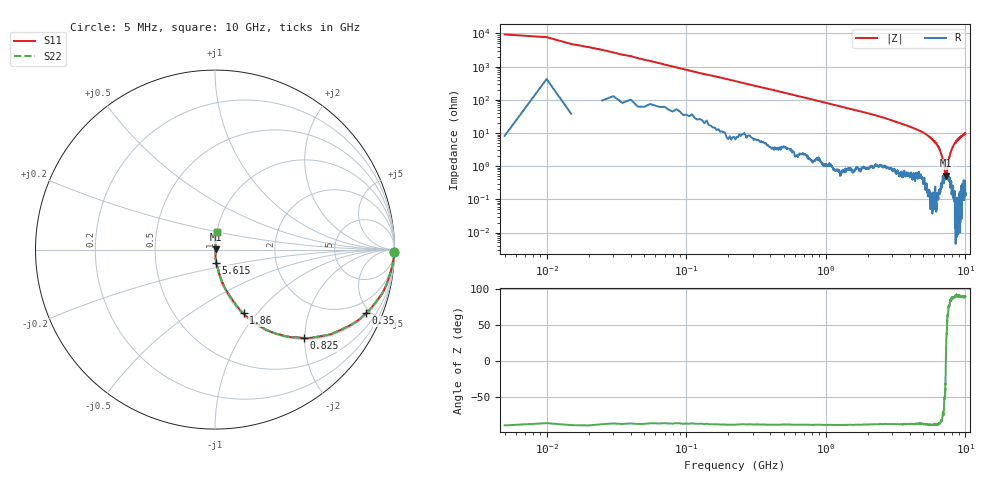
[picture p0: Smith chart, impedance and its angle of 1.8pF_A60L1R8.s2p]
! Amotech Co.,Ltd.
! http://www.amotech.co.kr/
! Part Number: A60L1R8
! These Parameters are Measured in Series Mode Connection
! Operation Temp=25[degC], DC Bias Voltage=0[V]
! Freq. Start=5[MHz] Stop=10[GHz], 2000[Steps]
! Date: Monday, July 14, 2020, 09:28:34
# GHZ S RI R 50.000000
!Freq.(Hz) S11(Real) S11(Imag) S21(Real) S21(Imag) S12(Real) S12(Imag) S22(Real) S22(Imag)
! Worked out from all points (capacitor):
!   2000 points, 5 MHz to 10 GHz, reference 50 ohm
!   read as one part in series: C = 1.98 pF near 55 MHz
!   lowest |Z| = 519 mohm at 7.28 GHz (marker M1)
!   series resonance near 7.248 GHz, so ESL is about 240 pH
!   S11 on the Smith chart (normalised r, x): 5 MHz: open; 350 MHz: 1.10, -4.72; 825 MHz: 1.03, -1.98; 1.86 GHz: 1.02, -0.85; 5.615 GHz: 1.00, -0.15; 10 GHz: 1.00, +0.20
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0.005  0.9999 -0.0107  0.000124 0.0107  0.000124 0.0107  0.9999 -0.0107
0.07  0.9881 -0.0851  0.0119 0.0851  0.0119 0.0851  0.9881 -0.0851
0.12  0.9728 -0.1447  0.0272 0.1447  0.0272 0.1447  0.9728 -0.1447
0.22  0.929 -0.2469  0.071 0.2469  0.071 0.2469  0.929 -0.2469
0.35  0.8422 -0.3538  0.1578 0.3538  0.1578 0.3538  0.8422 -0.3538
0.825  0.496 -0.4925  0.504 0.4925  0.504 0.4925  0.496 -0.4925
1.225  0.3042 -0.4546  0.6958 0.4546  0.6958 0.4546  0.3042 -0.4546
1.675  0.1894 -0.3826  0.8106 0.3826  0.8106 0.3826  0.1894 -0.3826
1.86  0.1591 -0.3546  0.8409 0.3546  0.8409 0.3546  0.1591 -0.3546
3.34  0.0437 -0.1917  0.9563 0.1917  0.9563 0.1917  0.0437 -0.1917
5.005  0.0132 -0.1004  0.9868 0.1004  0.9868 0.1004  0.0132 -0.1004
5.615  0.00605 -0.0728  0.9939 0.0728  0.9939 0.0728  0.00605 -0.0728
6.215  0.00285 -0.0478  0.9972 0.0478  0.9972 0.0478  0.00285 -0.0478
6.67  0.00336 -0.0257  0.9966 0.0257  0.9966 0.0257  0.00336 -0.0257
6.925  0.00441 -0.0136  0.9956 0.0136  0.9956 0.0136  0.00441 -0.0136
7.165  0.00419 -0.00366  0.9958 0.00366  0.9958 0.00366  0.00419 -0.00366
7.28  0.00487 0.0017  0.9951 -0.0017  0.9951 -0.0017  0.00487 0.0017
7.485  0.00592 0.0105  0.9941 -0.0105  0.9941 -0.0105  0.00592 0.0105
7.795  0.0032 0.0237  0.9968 -0.0237  0.9968 -0.0237  0.0032 0.0237
8.335  0.00327 0.0456  0.9967 -0.0456  0.9967 -0.0456  0.00327 0.0456
8.97  0.00493 0.0683  0.9951 -0.0683  0.9951 -0.0683  0.00493 0.0683
10  0.0108 0.0965  0.9892 -0.0965  0.9892 -0.0965  0.0108 0.0965
